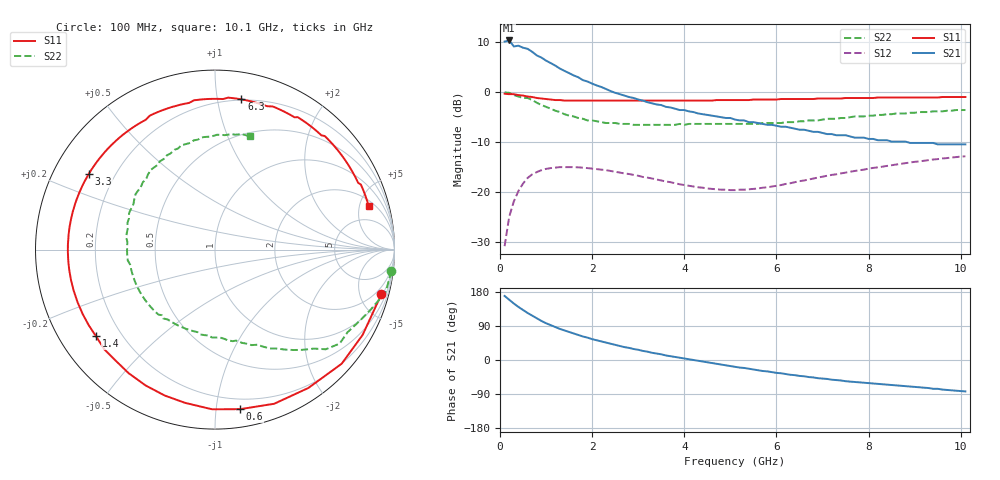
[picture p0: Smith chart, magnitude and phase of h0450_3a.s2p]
!HBFP-0450
!S and NOISE PARAMETERS at Vce=3V  Ic=1mA.  LAST UPDATED  09-04-98
# GHZ S MA R  50
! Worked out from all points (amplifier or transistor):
!   101 points, 100 MHz to 10.1 GHz, reference 50 ohm
!   highest |S21| = 10.3 dB at 200 MHz (marker M1)
!   |S21| within 3 dB of that: start of sweep to 801.9 MHz
!   unconditionally stable (mu >= 1): 3.321 GHz to end of sweep
!   at 1.7 GHz: K = 0.39, MSG = 9.0 dB, |S12| = -15.0 dB
!   at 5.1 GHz: K = 1.78, MAG = 1.9 dB, |S12| = -19.6 dB
!   at 10.1 GHz: K = 1.27, MAG = -1.9 dB, |S12| = -12.8 dB
!   lowest NFmin = 1.93 dB at 2 GHz
!   S11 on the Smith chart (normalised r, x): 100 MHz: 1.17, -7.41; 600 MHz: 0.12, -1.16; 1.4 GHz: 0.11, -0.32; 3.3 GHz: 0.11, +0.27; 6.3 GHz: 0.19, +1.17; 10.1 GHz: 2.56, +6.05
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0.1  0.96 -15.0  3.18 169.0  0.029 81.0  0.99 -7.0
0.2  0.95 -30.0  3.26 159.0  0.057 72.0  0.98 -14.0
0.3  0.95 -42.0  2.84 149.0  0.081 63.0  0.93 -21.0
0.4  0.93 -56.0  2.89 140.0  0.103 56.0  0.9 -26.0
0.6  0.9 -81.0  2.69 124.0  0.139 42.0  0.87 -37.0
0.8  0.87 -101.0  2.31 110.0  0.159 30.0  0.78 -45.0
0.9  0.86 -109.0  2.2 103.0  0.166 25.0  0.74 -49.0
1  0.85 -117.0  2.05 97.0  0.171 21.0  0.71 -52.0
1.2  0.83 -132.0  1.83 87.0  0.176 13.0  0.65 -58.0
1.4  0.82 -144.0  1.62 78.0  0.178 6.0  0.6 -64.0
1.8  0.82 -164.0  1.31 62.0  0.176 -5.0  0.54 -74.0
2.2  0.82 -179.0  1.12 49.0  0.168 -14.0  0.5 -84.0
2.5  0.82 171.0  0.98 40.0  0.16 -18.0  0.49 -92.0
3.3  0.82 149.0  0.77 19.0  0.137 -27.0  0.47 -112.0
3.5  0.82 144.0  0.74 15.0  0.131 -29.0  0.47 -117.0
5.1  0.83 107.0  0.53 -18.0  0.105 -24.0  0.48 -157.0
6.3  0.85 80.0  0.44 -39.0  0.123 -19.0  0.5 169.0
6.8  0.85 70.0  0.4 -46.0  0.137 -20.0  0.52 154.0
7.7  0.87 54.0  0.35 -58.0  0.163 -27.0  0.57 129.0
8.5  0.88 41.0  0.32 -66.0  0.186 -35.0  0.6 110.0
9.4  0.88 27.0  0.31 -76.0  0.212 -47.0  0.64 89.0
10.1  0.89 16.0  0.3 -83.0  0.228 -58.0  0.66 73.0
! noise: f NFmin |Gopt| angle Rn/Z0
1.8  1.94  0.66  150  0.12
2  1.93  0.69  161  0.08
2.5  2.28  0.73  -180  0.04
3.5  2.77  0.79  -149  0.26
4  3.11  0.81  -136  0.56
5  3.72  0.84  -111  1.72
5.5  3.91  0.87  -99  2.7
7  4.69  0.89  -67  6.48
8  4.97  0.89  -49  9.33
10  5.97  0.8  -19  11.54
